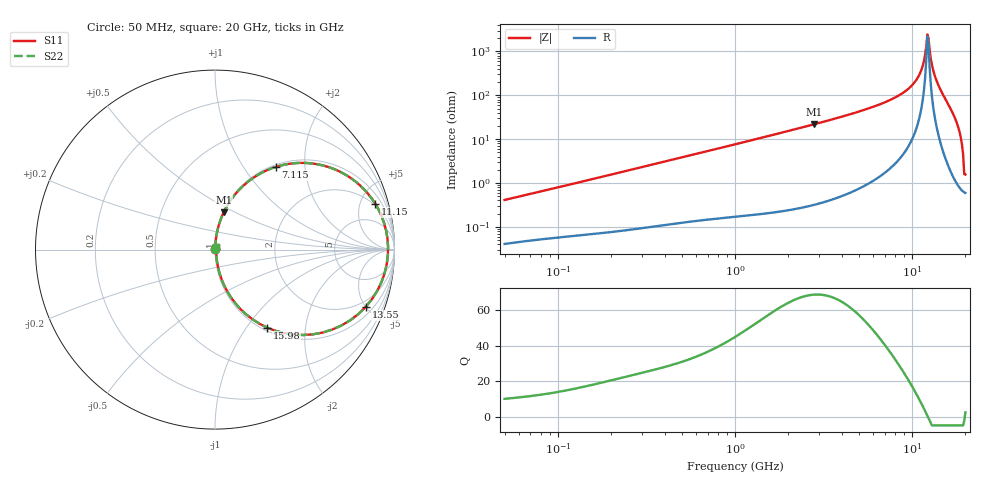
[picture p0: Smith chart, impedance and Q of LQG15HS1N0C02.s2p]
!Murata Part Number: LQG15HS1N0C02
!These Parameters are Measured in Series Mode Connection
!  o--[Z]--o
!Port1  Port2
!  o-------o
!Freq. Start=50[MHz] Stop=20[GHz], 401[Steps]
# Hz S RI R 50
!Freq.(Hz) S11(Real) S11(Imag) S21(Real) S21(Imag) S12(Real) S12(Imag) S22(Real) S22(Imag)
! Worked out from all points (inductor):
!   401 points, 50 MHz to 20 GHz, reference 50 ohm
!   read as one part in series: L = 1.29 nH near 51.52 MHz
!   highest Q = 68.8 at 2.811 GHz (marker M1), where L = 1.24 nH
!   self-resonance near 12.2 GHz
!   S11 on the Smith chart (normalised r, x): 50 MHz: 1.00, +0.01; 7.115 GHz: 1.04, +1.42; 11.15 GHz: 1.79, +6.65; 13.55 GHz: 1.52, -5.02; 15.98 GHz: 1.05, -1.26; 20 GHz: 1.01, +0.03
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5e7  0.000425 0.00409  0.9996 -0.00409  0.9996 -0.00409  0.000425 0.00409
1.364002e8  0.000761 0.0107  0.9992 -0.0107  0.9992 -0.0107  0.000761 0.0107
3.721004e8  0.00187 0.0286  0.9981 -0.0286  0.9981 -0.0286  0.00187 0.0286
1e9  0.00743 0.0754  0.9926 -0.0754  0.9926 -0.0754  0.00743 0.0754
2.728004e9  0.0459 0.2022  0.9541 -0.2022  0.9541 -0.2022  0.0459 0.2022
2.810964e9  0.0487 0.2082  0.9513 -0.2082  0.9513 -0.2082  0.0487 0.2082
4.89267e9  0.1501 0.3487  0.8499 -0.3487  0.8499 -0.3487  0.1501 0.3487
7.114996e9  0.3384 0.4607  0.6616 -0.4607  0.6616 -0.4607  0.3384 0.4607
7.442007e9  0.3745 0.4707  0.6255 -0.4707  0.6255 -0.4707  0.3745 0.4707
9.745021e9  0.6912 0.4364  0.3088 -0.4364  0.3088 -0.4364  0.6912 0.4364
1.115139e10  0.8928 0.2556  0.1072 -0.2556  0.1072 -0.2556  0.8928 0.2556
1.201863e10  0.9607 0.063  0.0393 -0.063  0.0393 -0.063  0.9607 0.063
1.220001e10  0.9642 0.0169  0.0358 -0.0169  0.0358 -0.0169  0.9642 0.0169
1.257102e10  0.957 -0.0804  0.043 0.0804  0.043 0.0804  0.957 -0.0804
1.295331e10  0.928 -0.1798  0.072 0.1798  0.072 0.1798  0.928 -0.1798
1.354865e10  0.8405 -0.3182  0.1595 0.3182  0.1595 0.3182  0.8405 -0.3182
1.460232e10  0.6014 -0.4616  0.3986 0.4616  0.3986 0.4616  0.6014 -0.4616
1.597544e10  0.2915 -0.4351  0.7085 0.4351  0.7085 0.4351  0.2915 -0.4351
1.721783e10  0.1149 -0.3009  0.8851 0.3009  0.8851 0.3009  0.1149 -0.3009
1.828096e10  0.0387 -0.1708  0.9613 0.1708  0.9613 0.1708  0.0387 -0.1708
1.88369e10  0.0187 -0.1063  0.9813 0.1063  0.9813 0.1063  0.0187 -0.1063
2e10  0.0061 0.0142  0.9939 -0.0142  0.9939 -0.0142  0.0061 0.0142
